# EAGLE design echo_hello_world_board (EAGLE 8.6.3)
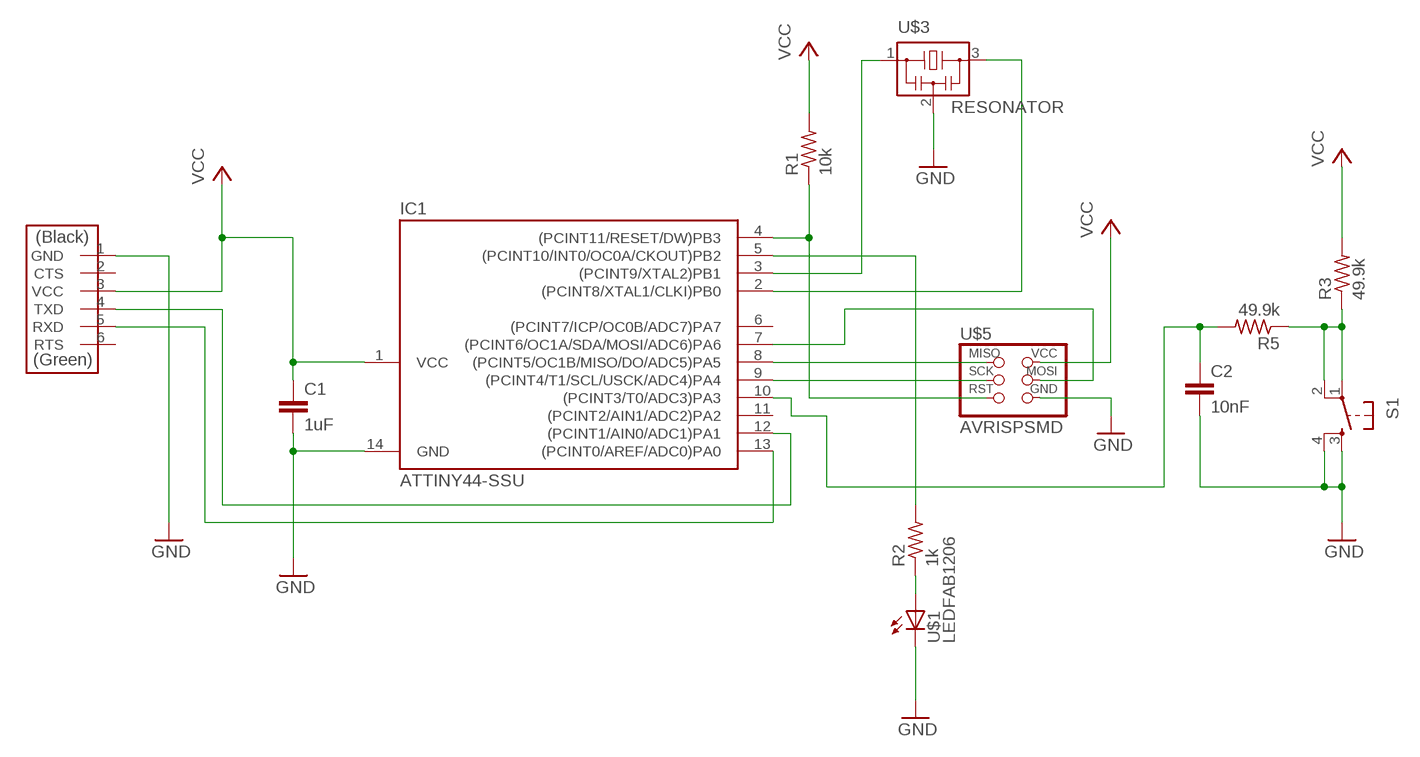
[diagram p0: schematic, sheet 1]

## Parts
C1  1uF  C-EUC3216  [C3216]
C2  10nF  C-EUC3216  [C3216]
IC1  ATTINY44-SSU  [SOIC14]
R1  10k  RES-US1206FAB  [R1206FAB]
R2  1k  RES-US1206FAB  [R1206FAB]
R3  49.9k  RES-US1206FAB  [R1206FAB]
R5  49.9k  RES-US1206FAB  [R1206FAB]
S1  6MM_SWITCH6MM_SWITCH  [6MM_SWITCH]
U$1  LEDFAB1206  [LED1206FAB]
U$2  FTDI-SMD-HEADER  [1X06SMD]
U$3  RESONATOR  [EFOBM]
U$5  AVRISPSMD  [2X03SMD]

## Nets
GND: C1.2 C2.2 IC1.14(GND) S1.3(S) S1.4(S1) U$1.2(C) U$2.1(GND) U$3.2 U$5.6(GND)
N$1: IC1.4((PCINT11/RESET/DW)PB3) R1.1 U$5.5(RST)
N$2: C2.1 IC1.10((PCINT3/T0/ADC3)PA3) R5.2
N$3: IC1.12((PCINT1/AIN0/ADC1)PA1) U$2.4(TXD)
N$4: IC1.13((PCINT0/AREF/ADC0)PA0) U$2.5(RXD)
N$5: IC1.5((PCINT10/INT0/OC0A/CKOUT)PB2) R2.2
N$6: R2.1 U$1.1(A)
N$7: IC1.3((PCINT9/XTAL2)PB1) U$3.1
N$8: IC1.8((PCINT5/OC1B/MISO/DO/ADC5)PA5) U$5.1(MISO)
N$9: IC1.9((PCINT4/T1/SCL/USCK/ADC4)PA4) U$5.3(SCK)
N$10: IC1.7((PCINT6/OC1A/SDA/MOSI/ADC6)PA6) U$5.4(MOSI)
N$11: R3.1 R5.1 S1.1(P) S1.2(P1)
N$13: IC1.2((PCINT8/XTAL1/CLKI)PB0) U$3.3
VCC: C1.1 IC1.1(VCC) R1.2 R3.2 U$2.3(VCC) U$5.2(VCC)
Unconnected: IC1.6((PCINT7/ICP/OC0B/ADC7)PA7) IC1.11((PCINT2/AIN1/ADC2)PA2) U$2.2(CTS) U$2.6(RTS)

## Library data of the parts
C1 C2 = rcl:C-EU: CAPACITOR, European symbol; SPICEPREFIX: C
IC1 = fab:ATTINY44
R1-R3 R5 = fab:RES-US: Resistor (US Symbol)
S1 = fab:6MM_SWITCH: OMRON SWITCH
U$1 = fab:LED: LED
U$2 = fab:FTDI-SMD-HEADER
U$3 = fab:RESONATOR
U$5 = fab:AVRISP

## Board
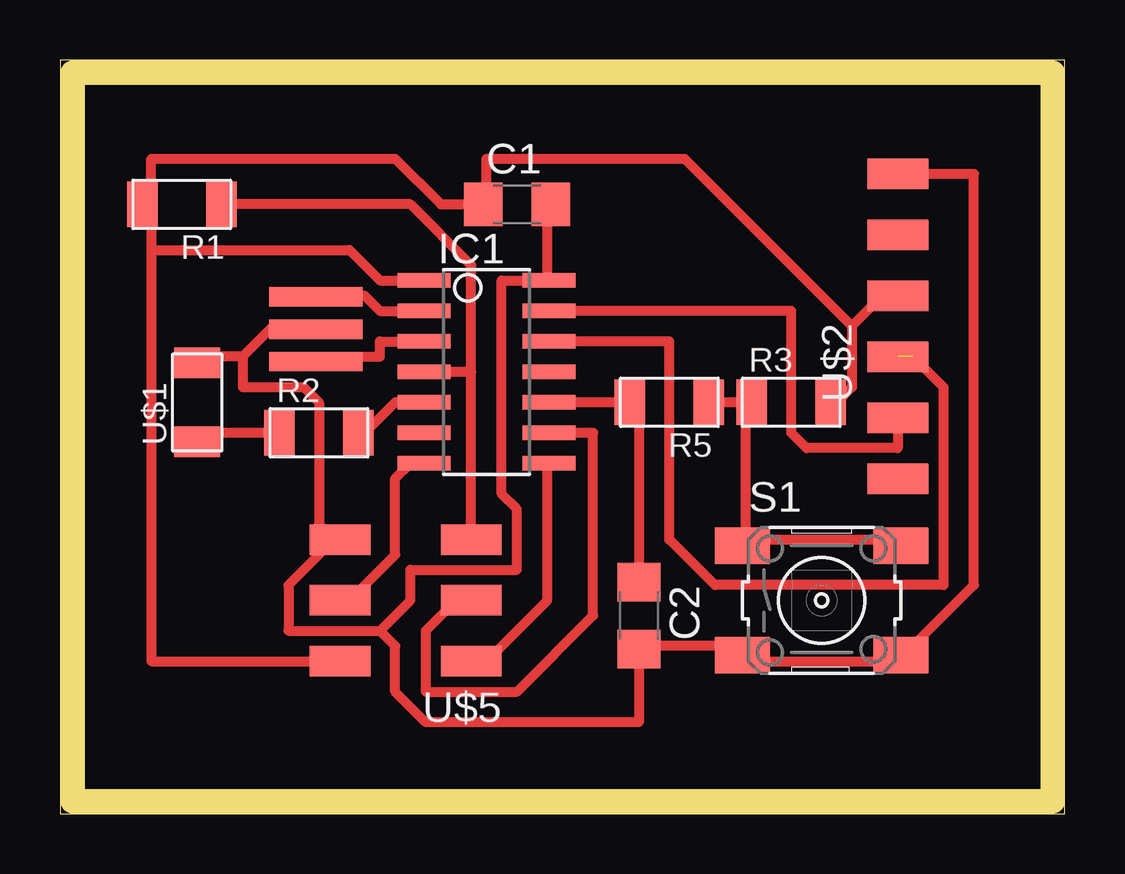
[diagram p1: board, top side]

Size 41.89 x 31.42 mm. Coordinates in mm from the lower left corner, seen from the top.
Outline: 0,0 41.89,0 41.89,31.42 0,31.42 0,0
Copper layers (1*16): Top 0.035mm / dielectric 1.5mm / Bottom 0.035mm
Design rules "default *": minimum track width 16mil, minimum drill 0.35mm, track to track 16mil, track to pad 16mil, pad to pad 16mil, via to via 16mil, smd to smd 16mil, copper to edge 40mil, drill to drill 16mil, minimum pad ring 10mil, minimum via ring 8mil, stop-mask expansion 4mil, vias tented up to drill 0mil, thermal gap 16mil
Milling: 4 lines

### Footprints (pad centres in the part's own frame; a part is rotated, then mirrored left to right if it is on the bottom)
C3216 = smd 1.6 x 1.8: 1 -1.4,0; 2 1.4,0
SOIC14 = smd 0.61 x 2.21: 1 -3.81,-2.603; 2 -2.54,-2.603; 3 -1.27,-2.603; 4 0,-2.603; 5 1.27,-2.603; 6 2.54,-2.603; 7 3.81,-2.603; 8 3.81,2.603; 9 2.54,2.603; 10 1.27,2.603; 11 0,2.603; 12 -1.27,2.603; 13 -2.54,2.603; 14 -3.81,2.603
R1206FAB = smd 1.27 x 1.905: 1 -1.651,0; 2 1.651,0
6MM_SWITCH = smd 2.286 x 1.524: 1 -3.302,2.286; 2 3.302,2.286; 3 -3.302,-2.286; 4 3.302,-2.286
LED1206FAB = smd 1.27 x 1.905: 1 -1.651,0; 2 1.651,0
1X06SMD = smd 2.54 x 1.27: 1 0,6.35; 2 0,3.81; 3 0,1.27; 4 0,-1.27; 5 0,-3.81; 6 0,-6.35
EFOBM = smd 0.8 x 3.9: 1 -1.35,0; 2 0,0; 3 1.35,0
2X03SMD = smd 2.54 x 1.27: 1 -2.54,2.54; 2 2.92,2.54; 3 -2.54,0; 4 2.92,0; 5 -2.54,-2.54; 6 2.92,-2.54

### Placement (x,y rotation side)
C1  19.05,25.4 0 top
C2  24.13,8.26 270 top
IC1  17.78,18.41 270 top
R1  5.08,25.4 180 top
R2  10.79,15.88 0 top
R3  30.48,17.14 0 top
R5  25.4,17.14 180 top
S1  31.75,8.89 0 top
U$1  5.71,17.14 90 top
U$2  34.92,20.32 0 top
U$3  10.67,20.19 90 top
U$5  14.61,8.89 180 top

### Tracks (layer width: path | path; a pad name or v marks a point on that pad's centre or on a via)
GND
  Top 0.406: 20.32,22.23 20.32,25.4 C1.2 | 7.62,19.05 5.71,19.05 U$1.2 | 7.62,19.05 8.89,20.32 10.16,20.32 U$3.2 | 11.43,11.43 10.79,12.06 10.79,17.14 10.16,17.78 7.62,17.78 7.62,19.05 | 20.32,22.23 18.41,22.23 18.41,13.34 19.05,12.7 19.05,10.16 14.61,10.16 14.61,8.89 13.34,7.62 | 13.34,7.62 9.53,7.62 9.53,9.53 11.43,11.43 | 20.32,22.23 IC1.14 | 11.43,11.43 U$5.6 | U$2.1 38.1,26.67 38.1,9.53 35.56,6.99 S1.4 34.92,6.35 28.57,6.35 S1.3 27.94,6.99 24.13,6.99 C2.2 24.13,3.81 15.24,3.81 13.97,5.08 13.97,6.99 13.34,7.62
N$1
  Top 0.406: R1.1 14.61,25.4 17.14,22.86 17.14,18.41 | U$5.5 17.14,18.41 | 17.14,18.41 IC1.4
N$2
  Top 0.406: C2.1 24.13,17.14 R5.2 IC1.10
N$3  (1 unrouted)
  Top 0.406: IC1.12 25.4,19.68 25.4,11.43 27.3,9.53 36.83,9.53 36.83,17.78 35.56,19.05
N$4
  Top 0.406: IC1.13 30.48,20.95 30.48,15.88 31.11,15.24 34.92,15.24 U$2.5
N$5
  Top 0.406: IC1.5 13.97,17.14 12.7,15.88 R2.2
N$6
  Top 0.406: R2.1 5.71,15.88 U$1.1
N$7
  Top 0.406: IC1.3 13.34,19.68 13.34,19.05 10.79,19.05 U$3.1
N$8
  Top 0.406: U$5.1 17.78,6.35 20.32,8.89 20.32,14.61 IC1.8
N$9
  Top 0.406: IC1.9 22.23,15.88 22.23,8.26 19.05,5.08 15.24,5.08 15.24,7.62 16.51,8.89 U$5.3
N$10
  Top 0.406: IC1.7 14.61,14.61 13.97,13.97 13.97,10.79 12.06,8.89 U$5.4
N$11
  Top 0.406: 28.57,17.14 R5.1 | 28.57,17.14 28.57,11.43 | 28.57,17.14 R3.1 | 28.57,11.43 34.92,11.43 S1.2 | 28.57,11.43 S1.1
N$13
  Top 0.406: IC1.2 13.34,20.95 12.7,21.59 10.79,21.59 U$3.3
VCC
  Top 0.406: 33.02,20.32 33.02,17.78 32.38,17.14 R3.2 | 33.02,20.32 34.29,21.59 U$2.3 | 3.81,25.4 3.81,27.3 13.97,27.3 15.88,25.4 C1.1 17.78,25.4 17.78,27.3 26.04,27.3 33.02,20.32 | IC1.1 13.34,22.23 12.06,23.5 3.81,23.5 | 3.81,25.4 3.81,23.5 | 3.81,25.4 R1.2 | U$5.2 3.81,6.35 3.81,23.5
